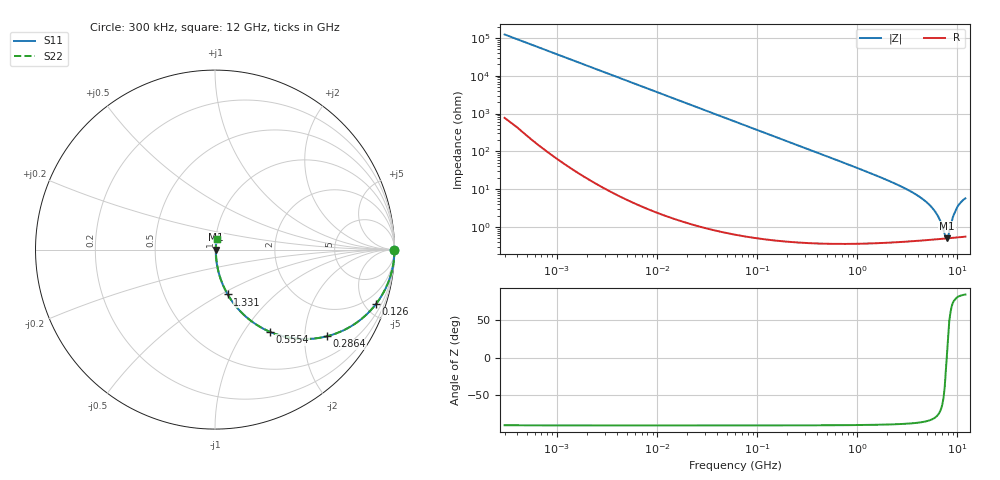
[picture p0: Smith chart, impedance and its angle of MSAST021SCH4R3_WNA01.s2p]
! MSAST021SCH4R3_WNA01  S-PARAMETER MODEL  ( General Type )
! Model Generated by TAIYO YUDEN Corporation (http://www.ty-top.com)
! Version 2.0
! TAIYO YUDEN Control No. 181101
! Copyright(c) 2015 TAIYO YUDEN CO.,LTD. All Rights Reserved.
! Product Description (link to TY-COMPAS)
! https://ds.yuden.co.jp/TYCOMPAS/or/detail?pn=MSAST021SCH4R3BWNA01&u=M
! Products Name : Multilayer Ceramic Capacitors
! Characteristics :
!  Capacitance : 4.3 pF , Rated Voltage : 25V , TCC : CH / C0H
!  Case Size : 0.25 x 0.125 / 0.0098 x 0.0049 [mm/inch] , Thickness : 0.125 / 0.0049 [mm/inch]
!  (Conditions: Temperature = 25 degC , DC Bias Current/Voltage = 0A / 0V)
! External Node Assignments :
!  1  o---| |---o  2
! GND o---------o GND
! Frequency Range : 0.3MHz  -  12000MHz  [ 401 STEP ]
# MHz S RI R 50
! Freq[MHz].  S11 Real  S11 Imag  S21 Real  S21 Imag  S12 Real  S12 Imag  S22 Real  S22 Imag
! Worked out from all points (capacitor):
!   401 points, 300 kHz to 12 GHz, reference 50 ohm
!   read as one part in series: C = 4.3 pF near 316.3 kHz
!   lowest |Z| = 505 mohm at 7.854 GHz (marker M1)
!   series resonance near 7.802 GHz, so ESL is about 97 pH
!   S11 on the Smith chart (normalised r, x): 300 kHz: open; 126 MHz: 1.01, -5.87; 286.4 MHz: 1.01, -2.58; 555.4 MHz: 1.01, -1.33; 1.331 GHz: 1.01, -0.54; 12 GHz: 1.01, +0.11
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0.3  1 -0.00081  5.72e-06 0.00081  5.72e-06 0.00081  1 -0.00081
1.769972  1 -0.00478  2.82e-05 0.00478  2.82e-05 0.00478  1 -0.00478
10.44266  0.9992 -0.0282  0.000814 0.0282  0.000814 0.0282  0.9992 -0.0282
60  0.9742 -0.1579  0.0258 0.1579  0.0258 0.1579  0.9742 -0.1579
125.9782  0.8957 -0.3048  0.1043 0.3048  0.1043 0.3048  0.8957 -0.3048
286.3882  0.6245 -0.4828  0.3755 0.4828  0.3755 0.4828  0.6245 -0.4828
353.9943  0.5212 -0.4978  0.4788 0.4978  0.4788 0.4978  0.5212 -0.4978
555.3718  0.3064 -0.4583  0.6936 0.4583  0.6936 0.4583  0.3064 -0.4583
848.5281  0.1587 -0.3613  0.8413 0.3613  0.8413 0.3613  0.1587 -0.3613
1331.232  0.0709 -0.2498  0.9291 0.2498  0.9291 0.2498  0.0709 -0.2498
2088.533  0.0299 -0.1589  0.9701 0.1589  0.9701 0.1589  0.0299 -0.1589
3642.919  0.0104 -0.0782  0.9896 0.0782  0.9896 0.0782  0.0104 -0.0782
5140.631  0.00615 -0.0401  0.9938 0.0401  0.9938 0.0401  0.00615 -0.0401
6188.031  0.0052 -0.0217  0.9948 0.0217  0.9948 0.0217  0.0052 -0.0217
6699.894  0.00501 -0.0141  0.995 0.0141  0.995 0.0141  0.00501 -0.0141
7448.838  0.00495 -0.00407  0.995 0.00407  0.995 0.00407  0.00495 -0.00407
7854.144  0.005 0.000533  0.995 -0.000533  0.995 -0.000533  0.005 0.000533
8281.503  0.00509 0.0058  0.9949 -0.0058  0.9949 -0.0058  0.00509 0.0058
8966.534  0.00544 0.0168  0.9946 -0.0168  0.9946 -0.0168  0.00544 0.0168
9708.23  0.00607 0.0284  0.9939 -0.0284  0.9939 -0.0284  0.00607 0.0284
10793.46  0.00735 0.0441  0.9926 -0.0441  0.9926 -0.0441  0.00735 0.0441
12000  0.00876 0.0563  0.9912 -0.0563  0.9912 -0.0563  0.00876 0.0563
